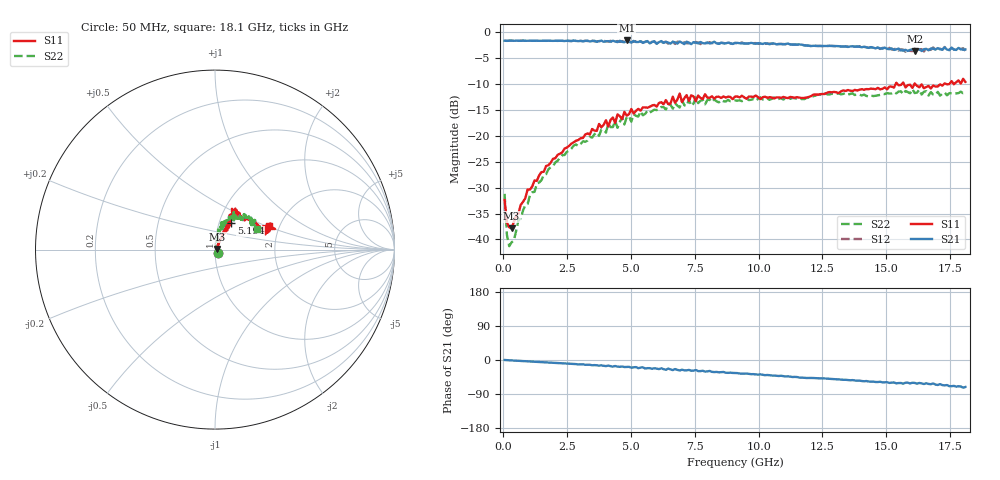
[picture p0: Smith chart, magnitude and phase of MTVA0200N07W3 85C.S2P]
! Network Analyzer HP8720D.06.14 Serial No. US36140669
!  7 Jul 2005  07:43:31
! Frequency  S11  S21  S12  S22
# HZ  S  DB R 50
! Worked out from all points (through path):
!   201 points, 50 MHz to 18.1 GHz, reference 50 ohm
!   highest |S21| = -1.63 dB at 4.833 GHz (marker M1); lowest = -3.7 dB at 16.11 GHz (marker M2)
!   group delay of S21, straight-line fit = 10.8 ps
!   lowest |S11| = -37.9 dB at 320.8 MHz (marker M3), VSWR 1.03, Z = 51.2 + j0.376 ohm
!   |S11| at or under -10 dB: start of sweep to 15.37 GHz; 15.69 GHz to 16.11 GHz (417.2 MHz wide, 2.62 % of centre); 16.13 GHz to 17.27 GHz (1.135 GHz wide, 6.8 % of centre)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
!   |S22| runs from -41.3 to -11.0 dB; largest |S21 - S12| = 0.047
!   S11 on the Smith chart (normalised r, x): 50 MHz: 1.03, -0.04; 5.194 GHz: 1.14, +0.35; 18.1 GHz: 1.77, +0.52
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5e7  -32.38 -51.2  -1.67 0.0  -1.66 0.0  -31.20 -50.1
1.4025e8  -36.74 -25.0  -1.71 -0.4  -1.70 -0.5  -39.13 -35.3
2.305e8  -37.62 -1.0  -1.67 -0.8  -1.66 -0.8  -41.29 -10.6
3.2075e8  -37.88 16.7  -1.66 -1.0  -1.68 -1.0  -40.56 18.6
9.525e8  -30.34 54.8  -1.69 -3.6  -1.67 -3.5  -33.14 70.4
1.3135e9  -28.70 61.5  -1.67 -4.9  -1.70 -5.0  -29.22 71.9
1.94525e9  -24.43 62.6  -1.71 -7.5  -1.70 -7.4  -25.90 77.1
3.1185e9  -20.42 62.7  -1.77 -11.4  -1.79 -11.9  -21.07 79.3
4.743e9  -15.39 61.4  -1.98 -18.6  -1.89 -17.4  -17.83 74.0
4.83325e9  -16.13 66.7  -1.63 -18.4  -1.88 -19.1  -16.38 68.0
5.19425e9  -15.21 58.6  -1.93 -18.7  -1.75 -19.2  -16.14 76.4
6.09675e9  -13.68 61.0  -1.95 -24.0  -1.83 -23.6  -14.88 66.5
6.7285e9  -13.65 67.2  -2.00 -23.9  -2.31 -24.9  -13.73 60.0
6.909e9  -11.86 63.7  -1.82 -27.7  -1.91 -25.5  -14.56 60.6
6.99925e9  -13.52 63.3  -2.08 -25.6  -2.27 -28.0  -13.11 60.7
7.17975e9  -12.17 67.5  -1.86 -27.4  -2.17 -25.8  -14.25 56.9
7.54075e9  -13.34 59.8  -2.06 -26.5  -1.92 -29.8  -12.60 63.5
9.075e9  -12.44 59.3  -2.12 -34.3  -2.09 -34.4  -13.19 53.8
1.21435e10  -12.07 43.8  -2.66 -47.5  -2.60 -47.5  -12.37 53.5
1.512175e10  -10.52 22.4  -3.31 -60.5  -3.05 -60.0  -11.85 44.2
1.61145e10  -9.92 18.5  -3.67 -60.5  -3.21 -60.8  -11.76 38.8
1.81e10  -9.61 23.4  -3.35 -71.2  -3.62 -71.1  -11.70 26.8
